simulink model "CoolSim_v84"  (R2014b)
settings: Solver=ode1  StartTime=0.0  StopTime=trun  FixedStep=dtmax  MaxStep=dtmax  MinStep=1e-6  RelTol=1e-4
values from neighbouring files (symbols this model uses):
  aperp_cond = l_cond*gappl_cond - l_cond*densfin_cond*thfin_cond*lfin_cond    (= 0.00397716486616)    [CoolSim_v84_ec_init.m]    (also in CoolSim_v84_mc_init.m)
  apin_txv = 1e-3^2/4*pi    (= 7.85398163397e-07)    [CoolSim_v84_ec_init.m]    (also in CoolSim_v84_mc_init.m)
  area_cabinint = 8.0    (= 8)    [CoolSim_v84_ec_init.m]    (also in CoolSim_v84_mc_init.m)
  area_cabinshell = 4.0    (= 4)    [CoolSim_v84_ec_init.m]    (also in CoolSim_v84_mc_init.m)
  aseat_txv = dball_txv^2/4*pi    (= 7.06858347058e-06)    [CoolSim_v84_ec_init.m]    (also in CoolSim_v84_mc_init.m)
  atop_txv = 400e-6    (= 0.0004)    [CoolSim_v84_ec_init.m]    (also in CoolSim_v84_mc_init.m)
  c08 = -5.8002206e+003    (= -5800.2206)    [CoolSim_v84_ec_init.m]    (also in CoolSim_v84_mc_init.m)
  c09 = 1.3914993    [CoolSim_v84_ec_init.m]    (also in CoolSim_v84_mc_init.m)
  c10 = -4.8640239E-02    (= -0.048640239)    [CoolSim_v84_ec_init.m]    (also in CoolSim_v84_mc_init.m)
  c11 = 4.1764768E-05    (= 4.1764768e-05)    [CoolSim_v84_ec_init.m]    (also in CoolSim_v84_mc_init.m)
  c12 = -1.4452093E-08    (= -1.4452093e-08)    [CoolSim_v84_ec_init.m]    (also in CoolSim_v84_mc_init.m)
  c13 = 6.5459673    [CoolSim_v84_ec_init.m]    (also in CoolSim_v84_mc_init.m)
  c1_comprmech = 0.8728    [CoolSim_v84_ec_init.m]    (also in CoolSim_v84_mc_init.m = 0.9)
  c2_comprmech = 0.1777    [CoolSim_v84_ec_init.m]    (also in CoolSim_v84_mc_init.m = 0)
  cv_air = 719.    (= 719)    [CoolSim_v84_ec_init.m]    (also in CoolSim_v84_mc_init.m)
  deltat = 2e-4    (= 0.0002)    [CoolSim_v84_ec_init.m]    (also in CoolSim_v84_mc_init.m)
  dh_evaptocomp = 0.0    (= 0)    [CoolSim_v84_ec_init.m]    (also in CoolSim_v84_mc_init.m)
  displ_compr = 33e-6    (= 3.3e-05)    [CoolSim_v84_ec_init.m]    (also in CoolSim_v84_mc_init.m = 0.0002)
  dp_blower = [0,  40., 160., 360.]    [CoolSim_v84_ec_init.m]    (also in CoolSim_v84_mc_init.m)
  dp_evaptocomp = 0.0    (= 0)    [CoolSim_v84_ec_init.m]    (also in CoolSim_v84_mc_init.m)
  dpair_cond = 2300.    (= 2300)    [CoolSim_v84_ec_init.m]    (also in CoolSim_v84_mc_init.m)
  dt_evapout = 0.5    [CoolSim_v84_ec_init.m]    (also in CoolSim_v84_mc_init.m)
  dt_thermostat = 0.2    [CoolSim_v84_ec_init.m]    (also in CoolSim_v84_mc_init.m)
  eff_blower = 0.12    [CoolSim_v84_ec_init.m]    (also in CoolSim_v84_mc_init.m)
  eff_fan = 0.15    [CoolSim_v84_ec_init.m]    (also in CoolSim_v84_mc_init.m)
  einitvec_cond1 = 10.*ones(1,nseg_cond1)    [CoolSim_v84_ec_init.m]    (also in CoolSim_v84_mc_init.m)
  einitvec_cond2 = 10.*ones(1,nseg_cond2)    [CoolSim_v84_ec_init.m]    (also in CoolSim_v84_mc_init.m)
  einitvec_evap1 = 10.*ones(1,nseg_evap1)    [CoolSim_v84_ec_init.m]    (also in CoolSim_v84_mc_init.m)
  einitvec_evap2a = 10.*ones(1,nseg_evap2)    [CoolSim_v84_ec_init.m]    (also in CoolSim_v84_mc_init.m)
  einitvec_evap2b = 10.*ones(1,nseg_evap2)    [CoolSim_v84_ec_init.m]    (also in CoolSim_v84_mc_init.m)
  einitvec_evap3 = 10.*ones(1,nseg_evap3)    [CoolSim_v84_ec_init.m]    (also in CoolSim_v84_mc_init.m)
  einitvec_evap4 = 10.*ones(1,nseg_evap4)    [CoolSim_v84_ec_init.m]    (also in CoolSim_v84_mc_init.m)
  f1_blowcontr = -0.7    [CoolSim_v84_ec_init.m]    (also in CoolSim_v84_mc_init.m)
  f1_comprcontr = -0.02    [CoolSim_v84_ec_init.m]    (also in CoolSim_v84_mc_init.m)
  f2_blowcontr = 0.005    [CoolSim_v84_ec_init.m]    (also in CoolSim_v84_mc_init.m)
  f2_comprcontr = 1./6.    (= 0.166666666667)    [CoolSim_v84_ec_init.m]    (also in CoolSim_v84_mc_init.m)
  fp_txv = (psetbulb_txv - pset_txv)*atop_txv - 15e5*aseat_txv    [CoolSim_v84_ec_init.m]    (also in CoolSim_v84_mc_init.m)
  h_lookuphvsps = h1    [CoolSim_v84_ec_init.m]    (also in CoolSim_v84_mc_init.m)
  hmax_heater = 8000.    (= 8000)    [CoolSim_v84_ec_init.m]    (also in CoolSim_v84_mc_init.m)
  htin_enginecomp = 0.0    (= 0)    [CoolSim_v84_ec_init.m]    (also in CoolSim_v84_mc_init.m; point_ec01.m; point_mc01.m)
  htin_solarintvstime = [htin_solarint htin_solarint]    [CoolSim_v84_ec_init.m]    (also in CoolSim_v84_mc_init.m; point_ec01.m = [300. 300.]; point_mc01.m = [300. 300.])
  htin_solarshellvstime = [htin_solarshell htin_solarshell]    [CoolSim_v84_ec_init.m]    (also in CoolSim_v84_mc_init.m; point_ec01.m = [1000. 1000.]; point_mc01.m = [1000. 1000.])
  htrans_cabinint = 25.    (= 25)    [CoolSim_v84_ec_init.m]    (also in CoolSim_v84_mc_init.m)
  htrans_cabinshell = 15.    (= 15)    [CoolSim_v84_ec_init.m]    (also in CoolSim_v84_mc_init.m)
  ifmech = 0.0    (= 0)    [CoolSim_v84_ec_init.m]    (also in CoolSim_v84_mc_init.m = 1)
  iinitvec_cond1 = 0.0*ones(1,nseg_cond1+1)    [CoolSim_v84_ec_init.m]    (also in CoolSim_v84_mc_init.m)
  iinitvec_cond2 = 0.0*ones(1,nseg_cond2+1)    [CoolSim_v84_ec_init.m]    (also in CoolSim_v84_mc_init.m)
  iinitvec_evap1 = 0.0*ones(1,nseg_evap1+1)    [CoolSim_v84_ec_init.m]    (also in CoolSim_v84_mc_init.m)
  iinitvec_evap2a = 0.0*ones(1,nseg_evap2+1)    [CoolSim_v84_ec_init.m]    (also in CoolSim_v84_mc_init.m)
  iinitvec_evap2b = 0.0*ones(1,nseg_evap2+1)    [CoolSim_v84_ec_init.m]    (also in CoolSim_v84_mc_init.m)
  iinitvec_evap3 = 0.0*ones(1,nseg_evap3+1)    [CoolSim_v84_ec_init.m]    (also in CoolSim_v84_mc_init.m)
  iinitvec_evap4 = 0.0*ones(1,nseg_evap4+1)    [CoolSim_v84_ec_init.m]    (also in CoolSim_v84_mc_init.m)
  init_memrestart = 2250.    (= 2250)    [CoolSim_v84_ec_init.m]    (also in CoolSim_v84_mc_init.m; reinit.m = memrestart(n,2))
  init_picontr1 = 0.23    [CoolSim_v84_ec_init.m]    (also in CoolSim_v84_mc_init.m; reinit.m = picontr1(n,2))
  init_picontr2 = 0.32    [CoolSim_v84_ec_init.m]    (also in CoolSim_v84_mc_init.m; reinit.m = picontr2(n,2))
  iseff_rpm_pr = [0.650   0.728   0.717   0.655   0.569;     0.570   0.682   0.700   0.637   0.536;     0.460   0.590   0.650   0.600   0.493;     0.290   0.496   0.618   0.575   0.450]    [CoolSim_v84_ec_init.m]    (also in CoolSim_v84_mc_init.m = [0.8490    0.8490    0.7829    0.7409    0.7065    0.6802   )
  k_cabinleakin = 1e-4    (= 0.0001)    [CoolSim_v84_ec_init.m]    (also in CoolSim_v84_mc_init.m)
  k_cabinleakout = 4e-4    (= 0.0004)    [CoolSim_v84_ec_init.m]    (also in CoolSim_v84_mc_init.m)
  k_ram = 0.1    [CoolSim_v84_ec_init.m]    (also in CoolSim_v84_mc_init.m)
  l_cabinsurf = 2.0    (= 2)    [CoolSim_v84_ec_init.m]    (also in CoolSim_v84_mc_init.m)
  md_comprmax = rpm_max/60.*displ_compr*0.975*27.8    (= 0.10435425)    [CoolSim_v84_ec_init.m]    (also in CoolSim_v84_mc_init.m = 0.63245)
  minitvec_cond1 = 1e-4*ones(1,nseg_cond1)    [CoolSim_v84_ec_init.m]    (also in CoolSim_v84_mc_init.m)
  minitvec_cond2 = 1e-4*ones(1,nseg_cond2)    [CoolSim_v84_ec_init.m]    (also in CoolSim_v84_mc_init.m)
  minitvec_evap1 = 1e-4*ones(1,nseg_evap1)    [CoolSim_v84_ec_init.m]    (also in CoolSim_v84_mc_init.m)
  minitvec_evap2a = 1e-4*ones(1,nseg_evap2)    [CoolSim_v84_ec_init.m]    (also in CoolSim_v84_mc_init.m)
  minitvec_evap2b = 1e-4*ones(1,nseg_evap2)    [CoolSim_v84_ec_init.m]    (also in CoolSim_v84_mc_init.m)
  minitvec_evap3 = 1e-4*ones(1,nseg_evap3)    [CoolSim_v84_ec_init.m]    (also in CoolSim_v84_mc_init.m)
  minitvec_evap4 = 1e-4*ones(1,nseg_evap4)    [CoolSim_v84_ec_init.m]    (also in CoolSim_v84_mc_init.m)
  mrefr_outrate = 0.2    [CoolSim_v84_ec_init.m]    (also in CoolSim_v84_mc_init.m)
  mrefr_targ = 0.48    [CoolSim_v84_ec_init.m]    (also in CoolSim_v84_mc_init.m)
  nc1 = 35.    (= 35)    [CoolSim_v84_ec_init.m]    (also in CoolSim_v84_mc_init.m)
  nc2 = 9.0    (= 9)    [CoolSim_v84_ec_init.m]    (also in CoolSim_v84_mc_init.m)
  ne1 = 7.    (= 7)    [CoolSim_v84_ec_init.m]    (also in CoolSim_v84_mc_init.m)
  ne2a = 5.    (= 5)    [CoolSim_v84_ec_init.m]    (also in CoolSim_v84_mc_init.m)
  ne2b = 15.    (= 15)    [CoolSim_v84_ec_init.m]    (also in CoolSim_v84_mc_init.m)
  ne3 = 12.    (= 12)    [CoolSim_v84_ec_init.m]    (also in CoolSim_v84_mc_init.m)
  ne4 = 15.    (= 15)    [CoolSim_v84_ec_init.m]    (also in CoolSim_v84_mc_init.m)
  onoff_fanonoffvstime = [1  1]    [CoolSim_v84_ec_init.m]    (also in CoolSim_v84_mc_init.m; point_ec01.m; point_mc01.m)
  onoffinit_cabin = 1.0    (= 1)    [CoolSim_v84_ec_init.m]    (also in CoolSim_v84_mc_init.m; reinit.m = onoff_cabin(n,2))
  onoffinit_evap = 1.0    (= 1)    [CoolSim_v84_ec_init.m]    (also in CoolSim_v84_mc_init.m; reinit.m = onoff_evap(n,2))
  p_ambient = 1.013e5    (= 101300)    [CoolSim_v84_ec_init.m]    (also in CoolSim_v84_mc_init.m)
  p_ambvstime = [p_ambient p_ambient]    [CoolSim_v84_ec_init.m]    (also in CoolSim_v84_mc_init.m; point_ec01.m = [101300. 101300.]; point_mc01.m = [101300. 101300.])
  p_lookup_tsatvsp = psat*1e5    [CoolSim_v84_ec_init.m]    (also in CoolSim_v84_mc_init.m)
  r_h2o = 461.5043    [CoolSim_v84_ec_init.m]    (also in CoolSim_v84_mc_init.m)
  rair = 287.    (= 287)    [CoolSim_v84_ec_init.m]    (also in CoolSim_v84_mc_init.m)
  rate_txv = 35e3    (= 35000)    [CoolSim_v84_ec_init.m]    (also in CoolSim_v84_mc_init.m)
  ratio_compr = 1.37    [CoolSim_v84_ec_init.m]    (also in CoolSim_v84_mc_init.m)
  rh_ambvstime = [rh_ambient rh_ambient]    [CoolSim_v84_ec_init.m]    (also in CoolSim_v84_mc_init.m; point_ec01.m = [50. 50.]; point_mc01.m = [50. 50.])
  rpm_max = 7000.    (= 7000)    [CoolSim_v84_ec_init.m]    (also in CoolSim_v84_mc_init.m)
  rpm_minmaxrat = 1500./7000.    (= 0.214285714286)    [CoolSim_v84_ec_init.m]    (also in CoolSim_v84_mc_init.m)
  rpm_rpmvstime = [1600,  1600]    [CoolSim_v84_ec_init.m]    (also in CoolSim_v84_mc_init.m; point_mc01.m)
  rpm_switchoff = rpm_max*rpm_minmaxrat*1.01    (= 1515)    [CoolSim_v84_ec_init.m]    (also in CoolSim_v84_mc_init.m)
  s_txv = 0.8e-3    (= 0.0008)    [CoolSim_v84_ec_init.m]    (also in CoolSim_v84_mc_init.m)
  scfm_blower = [0, 100., 200., 300.]    [CoolSim_v84_ec_init.m]    (also in CoolSim_v84_mc_init.m)
  set_steadystate = 0.0    (= 0)    [CoolSim_v84_ec_init.m]    (also in CoolSim_v84_mc_init.m)
  setting_blend = 0.0    (= 0)    [CoolSim_v84_ec_init.m]    (also in CoolSim_v84_mc_init.m; point_mc01.m)
  setting_blower = 3.0    (= 3)    [CoolSim_v84_ec_init.m]    (also in CoolSim_v84_mc_init.m; point_mc01.m)
  setting_recirc = -1.0    (= -1)    [CoolSim_v84_ec_init.m]    (also in CoolSim_v84_mc_init.m; point_mc01.m = 0.95)
  shape_cabinsurf = 0.5    [CoolSim_v84_ec_init.m]    (also in CoolSim_v84_mc_init.m)
  smin_txv = 1e-6    (= 1e-06)    [CoolSim_v84_ec_init.m]    (also in CoolSim_v84_mc_init.m)
  t_ambvstime = [t_ambient t_ambient]    [CoolSim_v84_ec_init.m]    (also in CoolSim_v84_mc_init.m; point_ec01.m = [303.16 303.16]; point_mc01.m = [303.16 303.16])
  t_lookup_tsatvsp = t1    [CoolSim_v84_ec_init.m]    (also in CoolSim_v84_mc_init.m)
  tairevapout_limit = 274.    (= 274)    [CoolSim_v84_ec_init.m]    (also in CoolSim_v84_mc_init.m)
  tairin_cond = 303.16    [CoolSim_v84_ec_init.m]    (also in CoolSim_v84_mc_init.m; point_ec01.m; point_mc01.m)
  tbulbinit_txv = 273.0    (= 273)    [CoolSim_v84_ec_init.m]    (also in CoolSim_v84_mc_init.m; reinit.m = tbulb_txv(n,2))
  tchar_txv = 0.1    [CoolSim_v84_ec_init.m]    (also in CoolSim_v84_mc_init.m)
  tdel_cycling = 5.0    (= 5)    [CoolSim_v84_ec_init.m]    (also in CoolSim_v84_mc_init.m)
  tdelinit_cycling = 1.0    (= 1)    [CoolSim_v84_ec_init.m]    (also in CoolSim_v84_mc_init.m; reinit.m = tdel_cycling1(n,2))
  tevap_target = 273.16+3.0    (= 276.16)    [CoolSim_v84_ec_init.m]    (also in CoolSim_v84_mc_init.m)
  thmass_cabinint = 2e5    (= 200000)    [CoolSim_v84_ec_init.m]    (also in CoolSim_v84_mc_init.m)
  thmass_cabinshell = 1e5    (= 100000)    [CoolSim_v84_ec_init.m]    (also in CoolSim_v84_mc_init.m)
  time0 = 0.0    (= 0)    [CoolSim_v84_ec_init.m]    (also in CoolSim_v84_mc_init.m; reinit.m = time11(n,2))
  time_ambvstime = [0 1e5]    [CoolSim_v84_ec_init.m]    (also in CoolSim_v84_mc_init.m; point_ec01.m; point_mc01.m)
  time_fanonoffvstime = [0 1e5]    [CoolSim_v84_ec_init.m]    (also in CoolSim_v84_mc_init.m; point_ec01.m; point_mc01.m)
  time_rpmvstime = [0,    10000]    [CoolSim_v84_ec_init.m]    (also in CoolSim_v84_mc_init.m; point_mc01.m)
  time_solarintvstime = [0 1e5]    [CoolSim_v84_ec_init.m]    (also in CoolSim_v84_mc_init.m; point_ec01.m; point_mc01.m)
  time_solarshellvstime = [0 1e5]    [CoolSim_v84_ec_init.m]    (also in CoolSim_v84_mc_init.m; point_ec01.m; point_mc01.m)
  time_velvstime = [0 1e5]    [CoolSim_v84_ec_init.m]    (also in CoolSim_v84_mc_init.m; point_ec01.m; point_mc01.m)
  tinit_cabinint = 313.16    [CoolSim_v84_ec_init.m]    (also in CoolSim_v84_mc_init.m; point_ec01.m; point_mc01.m; reinit.m = t_cabinint(n,2))
  tinit_cabinshell = 308.16    [CoolSim_v84_ec_init.m]    (also in CoolSim_v84_mc_init.m; point_ec01.m; point_mc01.m; reinit.m = t_cabinshell(n,2))
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undefined symbols (not defined in the file or in its folder): nseg
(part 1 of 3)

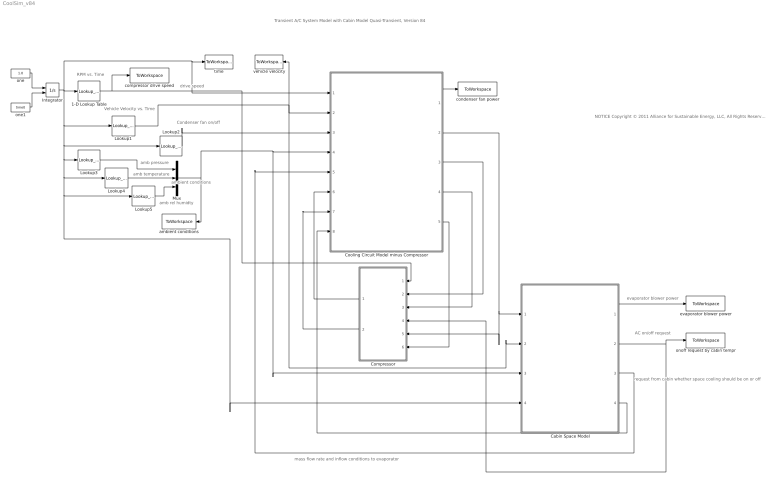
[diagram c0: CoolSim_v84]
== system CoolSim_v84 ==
  note: drive speed
  note: evaporator blower power
  note: RPM vs. Time
  note: Transient A/C System Model with Cabin Model Quasi-Transient, Version 84
  note: ambient conditions
  note: Vehicle Velocity vs. Time
  note: Condenser fan on/off
  note: amb pressure
  note: amb temperature
  note: amb rel humidty
  note: request from cabin whether space cooling should be on or off
  note: mass flow rate and inflow conditions to evaporator
  note: AC on/off request
  note: NOTICE Copyright © 2011 Alliance for Sustainable Energy, LLC, All Rights Reserved The CoolSim software (“ Software”) is being provided for internal, noncommercial purposes only and shall not be re-distributed. This Software was produced by Alliance for Sustainable Energy, LLC, (“Contactor”) under Contract No. DE-AC36-08GO28308 with the Department of Energy (“DOE”). For five (5) years from the date permission to assert copyright is obtained, the Government is granted for itself and others acting on its behalf a nonexclusive, paid-up, irrevocable worldwide license in this Software to reproduce, prepare derivative works, and perform publicly and display publicly, by or on behalf of the Government. There is provision for the possible extension of the term of this license. Subsequent to that period or any extension granted, the Government is granted for itself and others acting on its behalf a nonexclusive, paid-up, irrevocable worldwide license in this Software to reproduce, prepare derivative works, distribute copies to the public, perform publicly and display publicly, and to permit others to do so. The specific term of the license can be identified by inquiry made to Contractor or DOE. NEITHER THE UNITED STATES NOR THE UNITED STATES DEPARTMENT OF ENERGY, NOR ANY OF THEIR EMPLOYEES, MAKES ANY WARRANTY, EXPRESS OR IMPLIED, OR ASSUMES ANY LEGAL LIABILITY OR RESPONSIBILITY FOR THE ACCURACY, COMPLETENESS, OR USEFULNESS OF ANY DATA, APPARATUS, PRODUCT, OR PROCESS DISCLOSED, OR REPRESENTS THAT ITS USE WOULD NOT INFRINGE PRIVATELY OWNED RIGHTS.THIS SOFTWARE IS PROVIDED BY THE CONTRACTOR "AS IS" AND ANY EXPRESS OR IMPLIED WARRANTIES, INCLUDING BUT NOT LIMITED TO, THE IMPLIED WARRANTIES OF MERCHANTABILITY AND FITNESS FOR A PARTICULAR PURPOSE ARE EXPRESSLY DISCLAIMED. IN NO EVENT SHALL THE CONTRACTOR OR THE U.S. GOVERNMENT BE LIABLE FOR ANY SPECIAL, INDIRECT OR CONSEQUENTIAL DAMAGES OR ANY DAMAGES WHATSOEVER, INCLUDING BUT NOT LIMITED TO CLAIMS ASSOCIATED WITH THE LOSS OF DATA 
  1-D Lookup Table : Lookup_n-D  NumberOfTableDimensions=1  BreakpointsForDimension1=time_rpmvstime  Table=rpm_rpmvstime  RndMeth=Simplest
  Cabin Space Model : Subsystem
  Compressor : Subsystem
  Cooling Circuit Model minus Compressor : Subsystem
  Integrator : Integrator  InitialConditionSource=external
  Lookup1 : Lookup_n-D  NumberOfTableDimensions=1  BreakpointsForDimension1=time_velvstime  Table=vel_velvstime  RndMeth=Simplest
  Lookup2 : Lookup_n-D  NumberOfTableDimensions=1  BreakpointsForDimension1=time_fanonoffvstime  Table=onoff_fanonoffvstime  RndMeth=Simplest
  Lookup3 : Lookup_n-D  NumberOfTableDimensions=1  BreakpointsForDimension1=time_ambvstime  Table=p_ambvstime  RndMeth=Simplest
  Lookup4 : Lookup_n-D  NumberOfTableDimensions=1  BreakpointsForDimension1=time_ambvstime  Table=t_ambvstime  RndMeth=Simplest
  Lookup5 : Lookup_n-D  NumberOfTableDimensions=1  BreakpointsForDimension1=time_ambvstime  Table=rh_ambvstime  RndMeth=Simplest
  Mux : Mux  Inputs=3
  ambient conditions : ToWorkspace  VariableName=ambient  SampleTime=-1
  compressor drive speed : ToWorkspace  VariableName=rpm_drive1  SampleTime=-1
  condenser fan power : ToWorkspace  VariableName=power_condfan  SampleTime=-1
  evaporator blower power : ToWorkspace  VariableName=power_blower  SampleTime=-1
  one : Constant  Value=1.0
  one1 : Constant  Value=time0
  onoff request by cabin tempr : ToWorkspace  VariableName=onoff_cabin1  SampleTime=-1
  time : ToWorkspace  VariableName=time1  SampleTime=-1
  vehicle velocity : ToWorkspace  VariableName=velvehicle  SampleTime=-1
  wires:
  1-D Lookup Table/1 -> compressor drive speed/1, Compressor/1(rpm)
  Integrator/1 -> 1-D Lookup Table/1, Lookup1/1, Lookup4/1, Lookup5/1, Cabin Space Model/4(time1), Lookup3/1, Lookup2/1, time/1, Cooling Circuit Model minus Compressor/1(time1)
  one/1 -> Integrator/1
  one1/1 -> Integrator/2
  Lookup1/1 -> vehicle velocity/1, Cabin Space Model/2(vel_vechicle), Cooling Circuit Model minus Compressor/2(vel_vehicle)
  Mux/1 -> ambient conditions/1, Cooling Circuit Model minus Compressor/4(ambient), Cabin Space Model/3(ambient)
  Lookup3/1 -> Mux/1
  Lookup4/1 -> Mux/2
  Lookup5/1 -> Mux/3
  Lookup2/1 -> Cooling Circuit Model minus Compressor/3(fan)
  Cabin Space Model/1(pw_blower) -> evaporator blower power/1
  Cooling Circuit Model minus Compressor/1(power_cond_fan) -> condenser fan power/1
  Cooling Circuit Model minus Compressor/2(flowout_evap) -> Cabin Space Model/1(flowout_evap), Compressor/5(tevapout)
  Cabin Space Model/2(AC_request) -> onoff request by cabin tempr/1, Compressor/4(AC_request)
  Cabin Space Model/3(airevapin) -> Cooling Circuit Model minus Compressor/5(airinevap)
  Compressor/2(qd) -> Cooling Circuit Model minus Compressor/7(qdcompr)
  Cooling Circuit Model minus Compressor/3(pucompr) -> Compressor/2(ptrhu)
  Cooling Circuit Model minus Compressor/4(pdcompr) -> Compressor/3(ptrhd)
  Compressor/1(qu) -> Cooling Circuit Model minus Compressor/6(qucompr)
  Cabin Space Model/4(ambextras) -> Cooling Circuit Model minus Compressor/8(ambextras)
  Cooling Circuit Model minus Compressor/5(twallevap) -> Compressor/6(twallevap)

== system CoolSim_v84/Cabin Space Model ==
  note: mass flow rate from cabin to blower
  note: all air flow to blower
  note: total air inflow to cabin
  note: blower power use
  note: md, tempr, RH out evap
  note: fraction reheat request
  note: rho, h, ah ambient
  note: md, hd, ah
  note: md, hd, ah
  note: air mass flow rate to blower from cabin
  note: changed for mc02!!!
  flowout_evap : Inport
  vel_vechicle : Inport  Port=2
  ambient : Inport  Port=3
  time1 : Inport  Port=4
  airmix_volume02 CABIN : Subsystem
  cabin properties : ToWorkspace  VariableName=pcabin  SampleTime=-1
  calculate cabin heat load : Subsystem
  calculate air inflow to evap : Subsystem
  calculate cabin air inflow : Subsystem
  calculate desired settings : Subsystem
  calculate outflow from cabin : Subsystem
  evap airflow recirculated portion : ToWorkspace  VariableName=recirc  SampleTime=-1
  save data for reninitialization : Subsystem
  select pres : Fcn  Expr=u(1)
  zeros1 : Constant  Value=[vol_cabin, 0.0]
  pw_blower : Outport
  AC_request : Outport  Port=2
  airevapin : Outport  Port=3
  ambextras : Outport  Port=4
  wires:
  flowout_evap/1 -> calculate cabin air inflow/1(evapout)
  vel_vechicle/1 -> calculate cabin heat load/1(vveh)
  calculate desired settings/3(Blower) -> calculate air inflow to evap/2(blower)
  zeros1/1 -> airmix_volume02 CABIN/2("V, dVdt")
  airmix_volume02 CABIN/1(ptrh_mix) -> calculate desired settings/1(cabin), calculate air inflow to evap/1(cabin), calculate outflow from cabin/1(cabin), calculate cabin heat load/3(cabin), select pres/1, [pcabin], cabin properties/1
  calculate cabin air inflow/1(inflow) -> airmix_volume02 CABIN/1(qu)
  calculate outflow from cabin/1(outflow) -> airmix_volume02 CABIN/4(qd)
  ambient/1 -> calculate cabin heat load/2(ambient), calculate cabin air inflow/2(ambient), calculate outflow from cabin/2(ambient), calculate desired settings/2(ambient)
  calculate cabin heat load/1(htout) -> airmix_volume02 CABIN/3(Hout)
  calculate air inflow to evap/2(airinevap) -> airevapin/1
  calculate air inflow to evap/3(toevap) -> calculate outflow from cabin/3(toevap)
  calculate desired settings/4(Recirc) -> calculate air inflow to evap/3(recirc), evap airflow recirculated portion/1
  calculate desired settings/2(AC_on) -> AC_request/1
  calculate air inflow to evap/1(pwblower) -> pw_blower/1
  select pres/1 -> calculate cabin air inflow/3(pcabin)
  calculate desired settings/1(blend) -> calculate cabin air inflow/4(blend)
  [ambextras] -> calculate air inflow to evap/4(ambient), ambextras/1
  time1/1 -> calculate cabin heat load/4(time1)

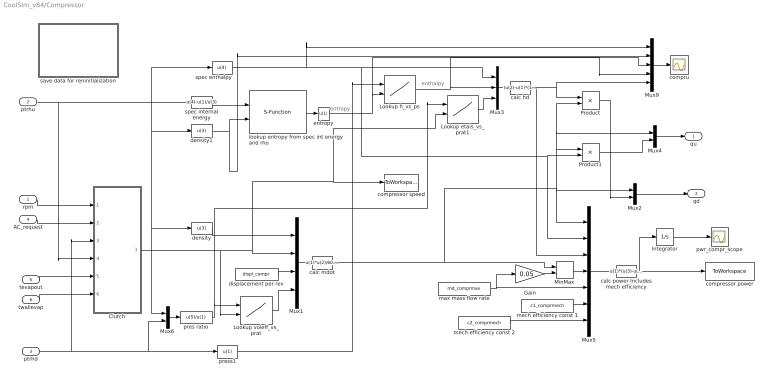
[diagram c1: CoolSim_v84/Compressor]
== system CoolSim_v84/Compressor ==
  note: enthalpy
  note: entropy
  rpm : Inport
  ptrhu : Inport  Port=2
  ptrhd : Inport  Port=3
  AC_request : Inport  Port=4
  tevapout : Inport  Port=5
  twallevap : Inport  Port=6
  Clutch : Subsystem
  Gain : Gain  Gain=0.05
  Integrator : Integrator
  Lookup etais_vs_prat1 : Lookup2D  RowIndex=voleff_prs  ColumnIndex=voleff_rpms  Table=iseff_rpm_pr  LookUpMeth=Interpolation-Use End Values
  Lookup h_vs_ps : Lookup2D  RowIndex=p_lookuphvsps  ColumnIndex=s_lookuphvsps  Table=h_lookuphvsps
  Lookup voleff_vs_prat : Lookup2D  RowIndex=voleff_prs  ColumnIndex=voleff_rpms  Table=voleff_rpm_pr  LookUpMeth=Interpolation-Use End Values
  MinMax : MinMax  Function=max  Inputs=2
  Mux1 : Mux
  Mux2 : Mux  Inputs=2
  Mux3 : Mux  Inputs=3
  Mux4 : Mux  Inputs=2
  Mux5 : Mux  Inputs=7
  Mux6 : Mux  Inputs=2
  Mux9 : Mux  Inputs=5
  Product : Product
  Product1 : Product
  calc hd : Fcn  Expr=(u(2)-u(1)*(1.0-u(3)))/u(3)
  calc mdot : Fcn  Expr=u(1)*u(2)/60.*u(3)*u(4)
  calc power Includes mech efficiency : Fcn  Expr=u(1)*(u(3)-u(2)) / (u(6)+u(7)*log( u(4)/u(5)))
  compressor power : ToWorkspace  VariableName=power_compr  SampleTime=-1
  compressor speed : ToWorkspace  VariableName=rpm_compr  SampleTime=-1
  compru : Scope
  density : Fcn  Expr=u(3)
  density1 : Fcn  Expr=u(3)
  displacement per rev : Constant  Value=displ_compr
  entropy : Fcn  Expr=u(1)
  lookup entropy from spec int energy and rho : S-Function  FunctionName=lookup_s_vs_urho  Parameters=1  EnableBusSupport=off
  max mass flow rate : Constant  Value=md_comprmax
  mech efficiency const 1 : Constant  Value=c1_comprmech
  mech efficiency const 2 : Constant  Value=c2_comprmech
  pres ratio : Fcn  Expr=u(5)/u(1)
  press1 : Fcn  Expr=u(1)
  pwr_compr_scope : Scope
  save data for reninitialization : Subsystem
  spec enthalpy : Fcn  Expr=u(4)
  spec internal energy : Fcn  Expr=u(4)-u(1)/u(3)
  qu : Outport
  qd : Outport  Port=2
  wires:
  ptrhu/1 -> Clutch/4(pucompr), spec internal energy/1, spec enthalpy/1, density/1, Mux6/1, density1/1
  density/1 -> Mux1/1
  Clutch/1(rpm) -> Mux1/2, compressor speed/1, Lookup etais_vs_prat1/2, Lookup voleff_vs_prat/2
  displacement per rev/1 -> Mux1/3
  Mux1/1 -> calc mdot/1
  ptrhd/1 -> press1/1, Mux6/2, Clutch/3(pdcompr)
  press1/1 -> Lookup h_vs_ps/1
  spec enthalpy/1 -> Mux3/1, Product1/2, Mux5/2, Mux9/1
  Lookup h_vs_ps/1 -> Mux9/4, Mux3/2
  Lookup etais_vs_prat1/1 -> Mux3/3
  Mux3/1 -> calc hd/1
  calc hd/1 -> Mux5/3, Product/1, Mux9/5
  calc mdot/1 -> Mux2/1, Product/2, Mux4/1, Product1/1, Mux5/1, MinMax/1
  Product/1 -> Mux2/2
  Mux2/1 -> qd/1
  Mux4/1 -> qu/1
  Product1/1 -> Mux4/2
  entropy/1 -> Lookup h_vs_ps/2, Mux9/3
  Mux6/1 -> pres ratio/1
  pres ratio/1 -> Lookup voleff_vs_prat/1, Lookup etais_vs_prat1/1
  Lookup voleff_vs_prat/1 -> Mux1/4
  lookup entropy from spec int energy and rho/1 -> entropy/1
  spec internal energy/1 -> lookup entropy from spec int energy and rho/1
  density1/1 -> lookup entropy from spec int energy and rho/2, Mux9/2
  Mux9/1 -> compru/1
  calc power Includes mech efficiency/1 -> Integrator/1, compressor power/1
  Integrator/1 -> pwr_compr_scope/1
  Mux5/1 -> calc power Includes mech efficiency/1
  mech efficiency const 2/1 -> Mux5/7
  max mass flow rate/1 -> Gain/1, Mux5/5
  Gain/1 -> MinMax/2
  MinMax/1 -> Mux5/4
  mech efficiency const 1/1 -> Mux5/6
  AC_request/1 -> Clutch/2(aconoff)
  rpm/1 -> Clutch/1(driverpm)
  tevapout/1 -> Clutch/5(tevapout)
  twallevap/1 -> Clutch/6(twallevap)

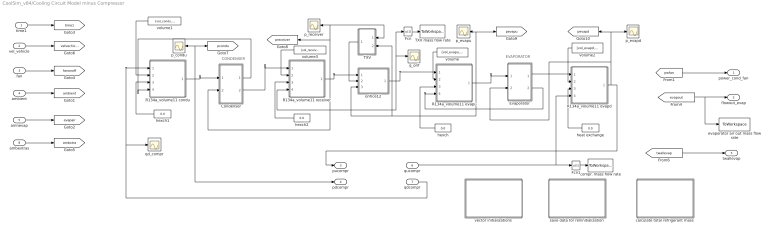
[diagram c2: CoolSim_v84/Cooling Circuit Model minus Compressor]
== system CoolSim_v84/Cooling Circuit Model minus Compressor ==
  note: CONDENSER
  note: EVAPORATOR
  time1 : Inport
  vel_vehicle : Inport  Port=2
  fan : Inport  Port=3
  ambient : Inport  Port=4
  airinevap : Inport  Port=5
  qucompr : Inport  Port=6
  qdcompr : Inport  Port=7
  ambextras : Inport  Port=8
  Condenser : Subsystem
  Evaporator : Subsystem
  Fcn : Fcn  Expr=u(1)
  Fcn1 : Fcn  Expr=u(1)
  R134a_volume11 condu : Subsystem
  R134a_volume11 evapd : Subsystem
  R134a_volume11 evapu : Subsystem
  R134a_volume11 receiver : Subsystem
  TXV : Subsystem
  TXV mass flow rate : ToWorkspace  VariableName=qorif  SampleTime=-1
  calculate total refrigerant mass : Subsystem
  compr. mass flow rate : ToWorkspace  VariableName=qcompr  SampleTime=-1
  evaporator air out mass flow rate : ToWorkspace  VariableName=mdaout_evap  SampleTime=-1
  heat exchange : Constant  Value=0.0
  hexch : Constant  Value=0.0
  hexch1 : Constant  Value=0.0
  hexch2 : Constant  Value=0.0
  orifice12 : Subsystem
  p_condu : Scope
  p_evapd : Scope
  p_evapu : Scope
  p_receiver : Scope
  q_orif : Scope
  qd_compr : Scope
  save data for reninitialization : Subsystem
  vector initializations : Subsystem
  volume : Constant  Value=[vol_evapu, 0]
  volume1 : Constant  Value=[vol_condu, 0]
  volume2 : Constant  Value=[vol_evapd, 0]
  volume3 : Constant  Value=[vol_receiver, 0]
  power_cond_fan : Outport
  flowout_evap : Outport  Port=2
  pucompr : Outport  Port=3
  pdcompr : Outport  Port=4
  twallevap : Outport  Port=5
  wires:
  R134a_volume11 condu/1(ptrh_mix) -> Condenser/1(ptrhu), p_condu/1, [pcondu], pdcompr/1
  orifice12/1(qmh) -> R134a_volume11 evapu/1(qu), q_orif/1, Fcn/1, R134a_volume11 receiver/4(qd)
  volume/1 -> R134a_volume11 evapu/2("V, dVdt")
  qucompr/1 -> R134a_volume11 evapd/4(qd), Fcn1/1
  volume1/1 -> R134a_volume11 condu/2("V, dVdt")
  qdcompr/1 -> R134a_volume11 condu/1(qu), qd_compr/1
  TXV/1(afr) -> orifice12/2(afrac)
  volume2/1 -> R134a_volume11 evapd/2("V, dVdt")
  R134a_volume11 evapd/1(ptrh_mix) -> Evaporator/2(ptrhd), p_evapd/1, [pevapd], pucompr/1
  heat exchange/1 -> R134a_volume11 evapd/3(Hout)
  R134a_volume11 evapu/1(ptrh_mix) -> Evaporator/1(ptrhu), p_evapu/1, [pevapu], orifice12/3(pTrhd), TXV/2(pd)
  hexch/1 -> R134a_volume11 evapu/3(Hout)
  R134a_volume11 receiver/1(ptrh_mix) -> orifice12/1(pTrhu), p_receiver/1, TXV/1(pu), [preceiver], Condenser/2(ptrhd)
  Condenser/1(qmhu) -> R134a_volume11 condu/4(qd)
  Condenser/2(qmhd) -> R134a_volume11 receiver/1(qu)
  volume3/1 -> R134a_volume11 receiver/2("V, dVdt")
  hexch2/1 -> R134a_volume11 receiver/3(Hout)
  hexch1/1 -> R134a_volume11 condu/3(Hout)
  Evaporator/1(qmhd) -> R134a_volume11 evapd/1(qu)
  Evaporator/2(qmhu) -> R134a_volume11 evapu/4(qd)
  [pwfan] -> power_cond_fan/1
  [evapout] -> flowout_evap/1, evaporator air out mass flow rate/1
  vel_vehicle/1 -> [velvechicle]
  ambient/1 -> [ambient]
  airinevap/1 -> [evapair]
  Fcn/1 -> TXV mass flow rate/1
  Fcn1/1 -> compr. mass flow rate/1
  fan/1 -> [fanonoff]
  ambextras/1 -> [ambxtra]
  [twallevap] -> twallevap/1
  time1/1 -> [time1]

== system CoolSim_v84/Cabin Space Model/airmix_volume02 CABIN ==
  note: p, T, rho, h, mh2o, rh, ah
  note: md_in, hd_in, ah_in
  note: md_out, hd_out, ah_out
  note: heat energy outflow rate
  note: volume, and time derivative of volume
  qu : Inport
  "V, dVdt" : Inport  Port=2
  Hout : Inport  Port=3
  qd : Inport  Port=4
  S-Function : S-Function  FunctionName=airmix_volume04  Parameters=vol0, mh2o0, p0, t0, rh0  EnableBusSupport=off
  ptrh_mix : Outport
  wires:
  qd/1 -> S-Function/4
  Hout/1 -> S-Function/3
  "V, dVdt"/1 -> S-Function/2
  S-Function/1 -> ptrh_mix/1
  qu/1 -> S-Function/1

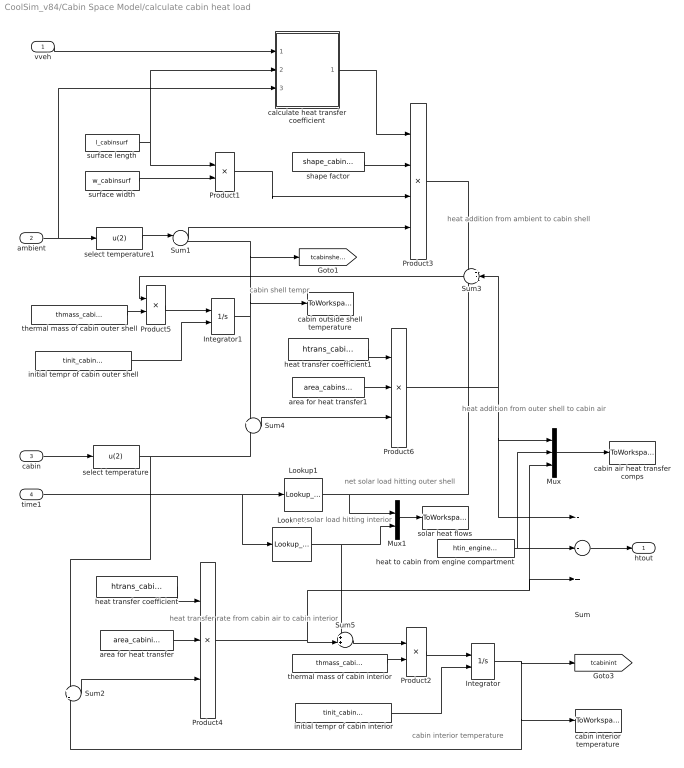
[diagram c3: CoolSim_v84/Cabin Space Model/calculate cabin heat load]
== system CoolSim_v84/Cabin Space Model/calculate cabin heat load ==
  note: heat addition from outer shell to cabin air
  note: cabin interior temperature
  note: heat transfer rate from cabin air to cabin interior
  note: cabin shell tempr
  note: heat addition from ambient to cabin shell
  note: net solar load hitting interior
  note: net solar load hitting outer shell
  vveh : Inport
  ambient : Inport  Port=2
  cabin : Inport  Port=3
  time1 : Inport  Port=4
  Integrator : Integrator  InitialConditionSource=external
  Integrator1 : Integrator  InitialConditionSource=external
  Lookup1 : Lookup_n-D  NumberOfTableDimensions=1  BreakpointsForDimension1=time_solarshellvstime  Table=htin_solarshellvstime  RndMeth=Simplest
  Lookup2 : Lookup_n-D  NumberOfTableDimensions=1  BreakpointsForDimension1=time_solarintvstime  Table=htin_solarintvstime  RndMeth=Simplest
  Mux : Mux  Inputs=3
  Mux1 : Mux  Inputs=2
  Product1 : Product
  Product2 : Product  Inputs=*/
  Product3 : Product  Inputs=4
  Product4 : Product  Inputs=3
  Product5 : Product  Inputs=*/
  Product6 : Product  Inputs=3
  Sum : Sum  Inputs=--+
  Sum1 : Sum  Inputs=|+-
  Sum2 : Sum  Inputs=+|-
  Sum3 : Sum  Inputs=+-+
  Sum4 : Sum  Inputs=+|-
  Sum5 : Sum  Inputs=++|
  area for heat transfer : Constant  Value=area_cabinint
  area for heat transfer1 : Constant  Value=area_cabinshell
  cabin air heat transfer comps : ToWorkspace  VariableName=hx_cabinair  SampleTime=-1
  cabin interior temperature : ToWorkspace  VariableName=tcabinint  SampleTime=-1
  cabin outside shell temperature : ToWorkspace  VariableName=tcabinshell  SampleTime=-1
  calculate heat transfer coefficient : Subsystem
  heat to cabin from engine compartment : Constant  Value=htin_enginecomp
  heat transfer coefficient : Constant  Value=htrans_cabinint
  heat transfer coefficient1 : Constant  Value=htrans_cabinshell
  initial tempr of cabin interior : Constant  Value=tinit_cabinint
  initial tempr of cabin outer shell : Constant  Value=tinit_cabinshell
  select temperature : Fcn  Expr=u(2)
  select temperature1 : Fcn  Expr=u(2)
  shape factor : Constant  Value=shape_cabinsurf
  solar heat flows : ToWorkspace  VariableName=htinsolar  SampleTime=-1
  surface length : Constant  Value=l_cabinsurf
  surface width : Constant  Value=w_cabinsurf
  thermal mass of cabin interior : Constant  Value=thmass_cabinint
  thermal mass of cabin outer shell : Constant  Value=thmass_cabinshell
  htout : Outport
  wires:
  ambient/1 -> select temperature1/1, calculate heat transfer coefficient/3(amb)
  cabin/1 -> select temperature/1
  select temperature1/1 -> Sum1/1
  select temperature/1 -> Sum2/1, Sum4/2
  heat to cabin from engine compartment/1 -> Sum/2, Mux/2
  Product3/1 -> Sum3/1
  Sum/1 -> htout/1
  shape factor/1 -> Product3/2
  vveh/1 -> calculate heat transfer coefficient/1(vveh)
  calculate heat transfer coefficient/1(h) -> Product3/1
  Product1/1 -> Product3/3
  surface width/1 -> Product1/2
  surface length/1 -> Product1/1, calculate heat transfer coefficient/2(Ingth)
  Integrator/1 -> [tcabinint], Sum2/2, cabin interior temperature/1
  Product2/1 -> Integrator/1
  thermal mass of cabin interior/1 -> Product2/2
  initial tempr of cabin interior/1 -> Integrator/2
  Sum2/1 -> Product4/3
  area for heat transfer/1 -> Product4/2
  heat transfer coefficient/1 -> Product4/1
  Sum1/1 -> Product3/4
  Product5/1 -> Integrator1/1
  thermal mass of cabin outer shell/1 -> Product5/2
  initial tempr of cabin outer shell/1 -> Integrator1/2
  Sum3/1 -> Product5/1
  area for heat transfer1/1 -> Product6/2
  heat transfer coefficient1/1 -> Product6/1
  Integrator1/1 -> Sum4/1, cabin outside shell temperature/1, Sum1/2, [tcabinshell]
  Sum4/1 -> Product6/3
  Product6/1 -> Sum/1, Mux/1, Sum3/2
  Sum5/1 -> Product2/1
  Product4/1 -> Sum5/2, Sum/3, Mux/3
  Lookup2/1 -> Mux1/2, Sum5/1
  Lookup1/1 -> Mux1/1, Sum3/3
  Mux1/1 -> solar heat flows/1
  Mux/1 -> cabin air heat transfer comps/1
  time1/1 -> Lookup2/1, Lookup1/1

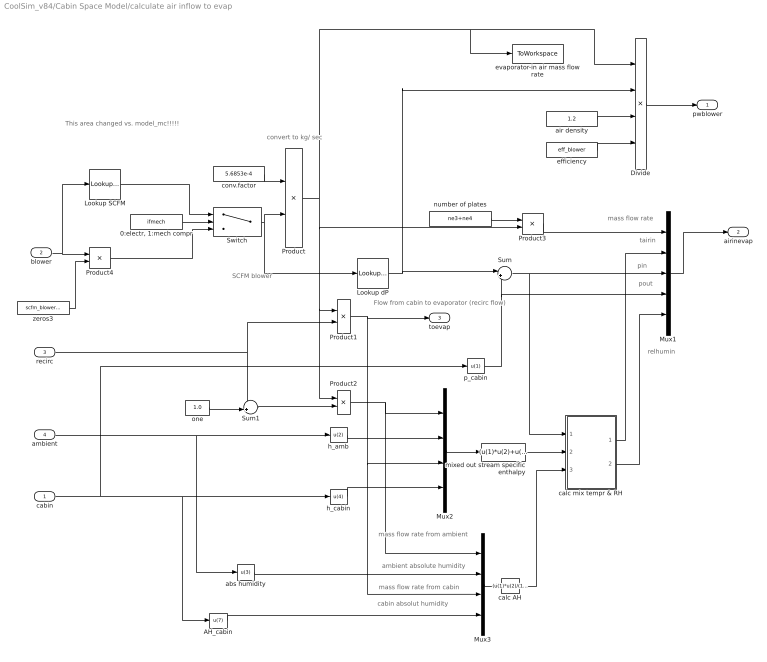
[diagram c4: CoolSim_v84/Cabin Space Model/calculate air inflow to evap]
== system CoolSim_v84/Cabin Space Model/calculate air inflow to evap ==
  note: mass flow rate
  note: tairin
  note: pin
  note: pout
  note: relhumin
  note: convert to kg/ sec
  note: Flow from cabin to evaporator (recirc flow)
  note: cabin absolut humidity
  note: ambient absolute humidity
  note: mass flow rate from ambient
  note: mass flow rate from cabin
  note: SCFM blower
  note: This area changed vs. model_mc!!!!!
  cabin : Inport
  blower : Inport  Port=2
  recirc : Inport  Port=3
  ambient : Inport  Port=4
  "0:electr, 1:mech compr" : Constant  Value=ifmech
  AH_cabin : Fcn  Expr=u(7)
  Divide : Product  Inputs=**//
  Lookup SCFM : Lookup_n-D  NumberOfTableDimensions=1  BreakpointsForDimension1=[0,1,2,3]  Table=scfm_blower  ExtrapMethod=Clip  RndMeth=Simplest
  Lookup dP : Lookup_n-D  NumberOfTableDimensions=1  BreakpointsForDimension1=scfm_blower  Table=dp_blower  ExtrapMethod=Clip  RndMeth=Simplest
  Mux1 : Mux  Inputs=5
  Mux2 : Mux
  Mux3 : Mux
  Product{,1..2,4} (4 alike) : Product
  Product3 : Product  Inputs=/*
  Sum : Sum  Inputs=|++
  Sum1 : Sum  Inputs=-+|
  Switch : Switch  Threshold=0.5
  abs humidity : Fcn  Expr=u(3)
  air density : Constant  Value=1.2
  calc AH : Fcn  Expr=(u(1)*u(2)/(1.+u(2))+u(3)*u(4)/(1.+u(4))) / (u(1)/(1.+u(2))+u(3)/(1.+u(4)))
  calc mix tempr & RH : Subsystem
  conv.factor : Constant  Value=5.6853e-4
  efficiency : Constant  Value=eff_blower
  evaporator-in air mass flow rate : ToWorkspace  VariableName=mdain_evap1  SampleTime=-1
  h_amb : Fcn  Expr=u(2)
  h_cabin : Fcn  Expr=u(4)
  mixed out stream specific enthalpy : Fcn  Expr=(u(1)*u(2)+u(3)*u(4))/(u(1)+u(3))
  number of plates : Constant  Value=ne3+ne4
  one : Constant  Value=1.0
  p_cabin : Fcn  Expr=u(1)
  zeros3 : Constant  Value=scfm_blower(4)
  pwblower : Outport
  airinevap : Outport  Port=2
  toevap : Outport  Port=3
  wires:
  cabin/1 -> h_cabin/1, AH_cabin/1, p_cabin/1
  recirc/1 -> Product1/2, Sum1/1
  ambient/1 -> abs humidity/1, h_amb/1
  mixed out stream specific enthalpy/1 -> calc mix tempr & RH/2(enth)
  Sum/1 -> Mux1/3, calc mix tempr & RH/1(press)
  Mux1/1 -> airinevap/1
  air density/1 -> Divide/3
  efficiency/1 -> Divide/4
  Divide/1 -> pwblower/1
  p_cabin/1 -> Mux1/4, Sum/2
  Lookup dP/1 -> Sum/1, Divide/2
  conv.factor/1 -> Product/1
  Product/1 -> evaporator-in air mass flow rate/1, Divide/1, Product1/1, Product2/1, Product3/2
  Product1/1 -> toevap/1, Mux3/3, Mux2/3
  one/1 -> Sum1/2
  h_cabin/1 -> Mux2/4
  Mux2/1 -> mixed out stream specific enthalpy/1
  Mux3/1 -> calc AH/1
  calc AH/1 -> calc mix tempr & RH/3(AH)
  calc mix tempr & RH/1(tempr) -> Mux1/2
  h_amb/1 -> Mux2/2
  calc mix tempr & RH/2(RH) -> Mux1/5
  AH_cabin/1 -> Mux3/4
  abs humidity/1 -> Mux3/2
  Sum1/1 -> Product2/2
  Product2/1 -> Mux2/1, Mux3/1
  Product3/1 -> Mux1/1
  number of plates/1 -> Product3/1
  zeros3/1 -> Product4/2
  blower/1 -> Product4/1, Lookup SCFM/1
  Switch/1 -> Product/2, Lookup dP/1
  "0:electr, 1:mech compr"/1 -> Switch/2
  Lookup SCFM/1 -> Switch/1
  Product4/1 -> Switch/3

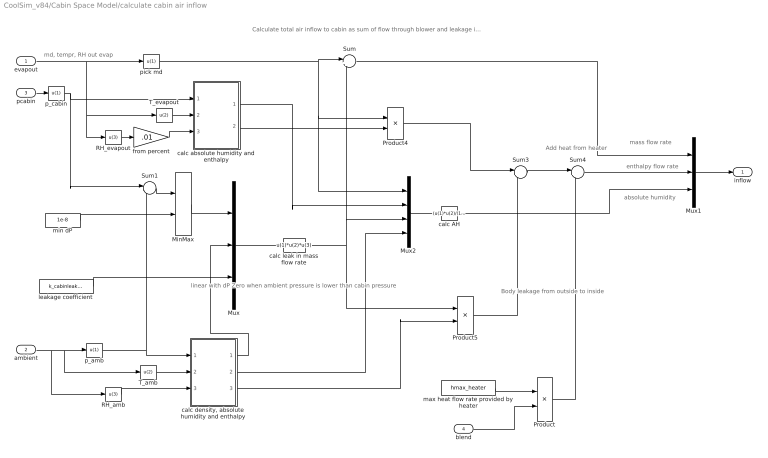
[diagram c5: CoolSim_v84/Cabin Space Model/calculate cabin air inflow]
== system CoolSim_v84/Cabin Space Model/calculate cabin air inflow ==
  note: Calculate total air inflow to cabin as sum of flow through blower and leakage into cabin from outside. Adjust enthalpy flow with heat added by heater
  note: md, tempr, RH out evap
  note: linear with dP Zero when ambient pressure is lower than cabin pressure
  note: absolute humidity
  note: mass flow rate
  note: enthalpy flow rate
  note: Add heat from heater
  note: Body leakage from outside to inside
  evapout : Inport
  ambient : Inport  Port=2
  pcabin : Inport  Port=3
  blend : Inport  Port=4
  MinMax : MinMax  Function=max  Inputs=2
  Mux : Mux  Inputs=3
  Mux1 : Mux  Inputs=3
  Mux2 : Mux
  Product : Product
  Product4 : Product
  Product5 : Product
  RH_amb : Fcn  Expr=u(3)
  RH_evapout : Fcn  Expr=u(3)
  Sum : Sum  Inputs=|++
  Sum1 : Sum  Inputs=|-+
  Sum3 : Sum  Inputs=|++
  Sum4 : Sum  Inputs=|++
  T_amb : Fcn  Expr=u(2)
  T_evapout : Fcn  Expr=u(2)
  calc AH : Fcn  Expr=(u(1)*u(2)/(1.+u(2))+u(3)*u(4)/(1.+u(4))) / (u(1)/(1.+u(2))+u(3)/(1.+u(4)))
  calc absolute humidity and enthalpy : Subsystem
  "calc density, absolute humidity and enthalpy" : Subsystem
  calc leak in mass flow rate : Fcn  Expr=u(1)*u(2)*u(3)
  from percent : Gain  Gain=.01
  leakage coefficient : Constant  Value=k_cabinleakin
  max heat flow rate provided by heater : Constant  Value=hmax_heater
  min dP : Constant  Value=1e-8
  p_amb : Fcn  Expr=u(1)
  p_cabin : Fcn  Expr=u(1)
  pick md : Fcn  Expr=u(1)
  inflow : Outport
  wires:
  evapout/1 -> T_evapout/1, RH_evapout/1, pick md/1
  blend/1 -> Product/2
  max heat flow rate provided by heater/1 -> Product/1
  pcabin/1 -> p_cabin/1
  T_evapout/1 -> calc absolute humidity and enthalpy/2(tempr)
  p_cabin/1 -> Sum1/1, calc absolute humidity and enthalpy/1(press)
  RH_evapout/1 -> from percent/1
  ambient/1 -> p_amb/1, T_amb/1, RH_amb/1
  p_amb/1 -> "calc density, absolute humidity and enthalpy"/1(press), Sum1/2
  T_amb/1 -> "calc density, absolute humidity and enthalpy"/2(tempr)
  RH_amb/1 -> "calc density, absolute humidity and enthalpy"/3(RH)
  calc leak in mass flow rate/1 -> Product5/1, Mux2/3, Sum/2
  Mux1/1 -> inflow/1
  Sum1/1 -> MinMax/1
  min dP/1 -> MinMax/2
  MinMax/1 -> Mux/1
  Mux/1 -> calc leak in mass flow rate/1
  Sum/1 -> Mux1/1
  calc absolute humidity and enthalpy/2(enth) -> Product4/2
  Product5/1 -> Sum3/2
  Product4/1 -> Sum3/1
  Sum4/1 -> Mux1/2
  Sum3/1 -> Sum4/1
  Product/1 -> Sum4/2
  "calc density, absolute humidity and enthalpy"/3(enth) -> Product5/2
  "calc density, absolute humidity and enthalpy"/1(dens) -> Mux/2
  calc absolute humidity and enthalpy/1(AH) -> Mux2/2
  "calc density, absolute humidity and enthalpy"/2(AH) -> Mux2/4
  Mux2/1 -> calc AH/1
  calc AH/1 -> Mux1/3
  leakage coefficient/1 -> Mux/3
  pick md/1 -> Sum/1, Product4/1, Mux2/1
  from percent/1 -> calc absolute humidity and enthalpy/3(RH)

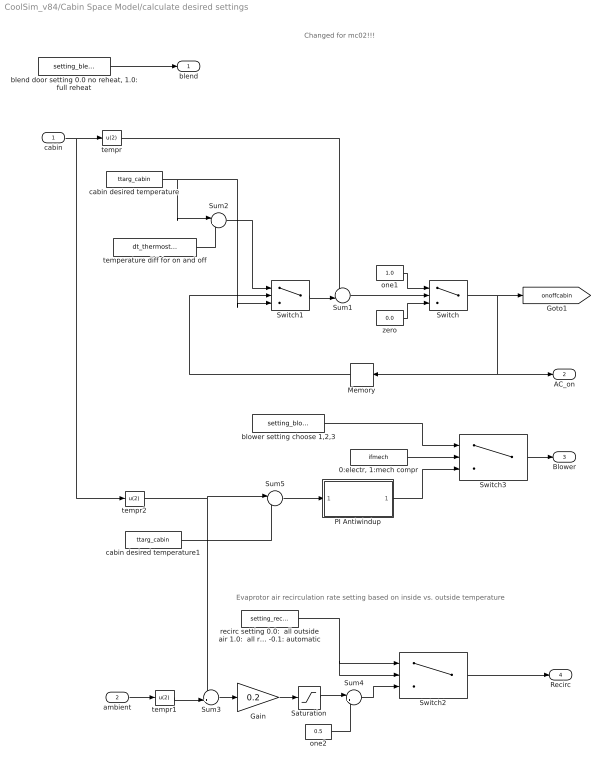
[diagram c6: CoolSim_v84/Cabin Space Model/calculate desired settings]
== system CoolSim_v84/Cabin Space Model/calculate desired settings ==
  note: Changed for mc02!!!
  note: Evaprotor air recirculation rate setting based on inside vs. outside temperature
  cabin : Inport
  ambient : Inport  Port=2
  "0:electr, 1:mech compr" : Constant  Value=ifmech
  Gain : Gain  Gain=0.2
  Memory : Memory  X0=onoffinit_cabin
  PI Antiwindup : Subsystem
  Saturation : Saturate  UpperLimit=0.45  LowerLimit=-0.45
  Sum1 : Sum  Inputs=+-|
  Sum2 : Sum  Inputs=|+-
  Sum3 : Sum  Inputs=-+|
  Sum4 : Sum  Inputs=|++
  Sum5 : Sum  Inputs=|-+
  Switch : Switch
  Switch1 : Switch  Threshold=0.5
  Switch2 : Switch  Threshold=-0.05
  Switch3 : Switch  Threshold=0.5
  "blend door setting 0.0 no reheat, 1.0: full reheat" : Constant  Value=setting_blend
  blower setting choose 1,2,3 : Constant  Value=setting_blower
  cabin desired temperature : Constant  Value=ttarg_cabin
  cabin desired temperature1 : Constant  Value=ttarg_cabin
  one1 : Constant  Value=1.0
  one2 : Constant  Value=0.5
  recirc setting 0.0:  all outside air 1.0:  all recirc air < -0.1: automatic : Constant  Value=setting_recirc
  temperature diff for on and off : Constant  Value=dt_thermostat
  tempr : Fcn  Expr=u(2)
  tempr1 : Fcn  Expr=u(2)
  tempr2 : Fcn  Expr=u(2)
  zero : Constant  Value=0.0
  blend : Outport
  AC_on : Outport  Port=2
  Blower : Outport  Port=3
  Recirc : Outport  Port=4
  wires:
  "0:electr, 1:mech compr"/1 -> Switch3/2
  cabin/1 -> tempr/1, tempr2/1
  "blend door setting 0.0 no reheat, 1.0: full reheat"/1 -> blend/1
  tempr/1 -> Sum1/1
  cabin desired temperature/1 -> Sum2/1, Switch1/3
  Sum2/1 -> Switch1/1
  Switch/1 -> Memory/1, AC_on/1, [onoffcabin]
  Sum1/1 -> Switch/2
  Switch1/1 -> Sum1/2
  Memory/1 -> Switch1/2
  one1/1 -> Switch/1
  zero/1 -> Switch/3
  temperature diff for on and off/1 -> Sum2/2
  Sum3/1 -> Gain/1
  recirc setting 0.0:  all outside air 1.0:  all recirc air < -0.1: automatic/1 -> Switch2/2, Switch2/1
  tempr1/1 -> Sum3/2
  ambient/1 -> tempr1/1
  Gain/1 -> Saturation/1
  Sum4/1 -> Switch2/3
  Saturation/1 -> Sum4/1
  one2/1 -> Sum4/2
  Switch2/1 -> Recirc/1
  tempr2/1 -> Sum5/1, Sum3/1
  cabin desired temperature1/1 -> Sum5/2
  Sum5/1 -> PI Antiwindup/1(err)
  blower setting choose 1,2,3/1 -> Switch3/1
  PI Antiwindup/1(cntrl) -> Switch3/3
  Switch3/1 -> Blower/1

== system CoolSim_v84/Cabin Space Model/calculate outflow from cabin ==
  note: Linear with dP Zero when ambient pressure is greater than cabin pressure
  note: md_out
  note: hd_out
  note: AH_out
  note: Calculate total air outflow from cabin, as the sum of recirc air outflow and leakage outflow
  cabin : Inport
  ambient : Inport  Port=2
  toevap : Inport  Port=3
  MinMax : MinMax  Function=max  Inputs=2
  Mux : Mux  Inputs=3
  Mux1 : Mux  Inputs=3
  Product1 : Product
  Sum : Sum  Inputs=|++
  Sum1 : Sum  Inputs=|+-
  calc leak out mass flow rate : Fcn  Expr=u(1)*u(2)*u(3)
  leakage effective flow area : Constant  Value=k_cabinleakout
  min dP : Constant  Value=1e-8
  pick AH : Fcn  Expr=u(7)
  pick density : Fcn  Expr=u(1)
  pick enthalpy : Fcn  Expr=u(4)
  pick press : Fcn  Expr=u(1)
  pick press1 : Fcn  Expr=u(1)
  outflow : Outport
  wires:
  cabin/1 -> pick enthalpy/1, pick AH/1, pick press/1
  ambient/1 -> pick press1/1
  calc leak out mass flow rate/1 -> Sum/2
  Sum/1 -> Product1/1, Mux1/1
  pick enthalpy/1 -> Product1/2
  Mux1/1 -> outflow/1
  Product1/1 -> Mux1/2
  pick AH/1 -> Mux1/3
  Sum1/1 -> MinMax/1
  min dP/1 -> MinMax/2
  MinMax/1 -> Mux/1
  Mux/1 -> calc leak out mass flow rate/1
  pick press/1 -> Sum1/1
  pick press1/1 -> Sum1/2
  toevap/1 -> Sum/1
  leakage effective flow area/1 -> Mux/3
  [ambextras] -> pick density/1
  pick density/1 -> Mux/2

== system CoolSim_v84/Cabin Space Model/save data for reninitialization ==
  onoff_cabin : Scope
  p_cabin : Scope
  picontr1 : Scope
  t_cabinint : Scope
  t_cabinshell : Scope
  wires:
  [pcabin] -> p_cabin/1
  [onoffcabin] -> onoff_cabin/1
  [tcabinint] -> t_cabinint/1
  [tcabinshell] -> t_cabinshell/1
  [picontr1] -> picontr1/1

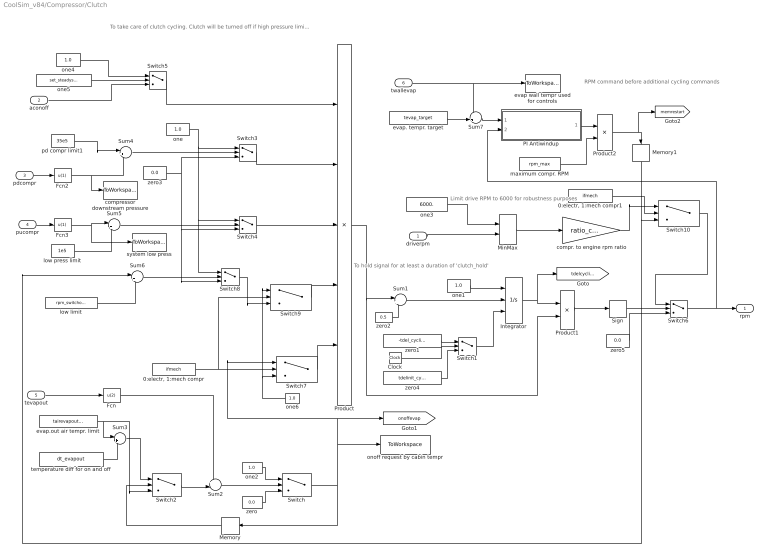
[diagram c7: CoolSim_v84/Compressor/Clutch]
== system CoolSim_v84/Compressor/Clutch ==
  note: To hold signal for at least a duration of 'clutch_hold'
  note: To take care of clutch cycling. Clutch will be turned off if high pressure limit, low pressure limit, or evaporator air temperature out low limit triggers it. It also turns off if temperature in the cabin drops below ttarg_cabin
  note: Limit drive RPM to 6000 for robustness purposes
  note: RPM command before additional cycling commands
  driverpm : Inport
  aconoff : Inport  Port=2
  pdcompr : Inport  Port=3
  pucompr : Inport  Port=4
  tevapout : Inport  Port=5
  twallevap : Inport  Port=6
  "0:electr, 1:mech compr" : Constant  Value=ifmech
  "0:electr, 1:mech compr1" : Constant  Value=ifmech
  Clock : Clock
  Fcn : Fcn  Expr=u(2)
  Fcn2 : Fcn  Expr=u(1)
  Fcn3 : Fcn  Expr=u(1)
  Integrator : Integrator  ExternalReset=falling  InitialConditionSource=external
  Memory : Memory  X0=onoffinit_evap
  Memory1 : Memory  X0=init_memrestart
  MinMax : MinMax  Inputs=2
  PI Antiwindup : Subsystem
  Product : Product  Inputs=5
  Product1 : Product
  Product2 : Product
  Sign : Signum
  Sum{1,3..6} (5 alike) : Sum  Inputs=|+-
  Sum2 : Sum  Inputs=+-|
  Sum7 : Sum  Inputs=-+|
  Switch : Switch
  Switch1 : Switch  Threshold=1e-8
  Switch{2,5..7,9..10} (6 alike) : Switch  Threshold=0.5
  Switch3 : Switch  Threshold=0.0
  Switch4 : Switch  Threshold=0.0
  Switch8 : Switch  Threshold=0.0
  compr. to engine rpm ratio : Gain  Gain=ratio_compr
  compressor downstream pressure : ToWorkspace  VariableName=pdcompr  SampleTime=-1
  evap wall tempr used for controls : ToWorkspace  VariableName=tevapwall  SampleTime=-1
  evap. tempr. target : Constant  Value=tevap_target
  evap.out air tempr. limit : Constant  Value=tairevapout_limit
  low limit : Constant  Value=rpm_switchoff
  low press limit : Constant  Value=1e5
  maximum compr. RPM : Constant  Value=rpm_max
  one{,1..2,4,6} (5 alike) : Constant  Value=1.0
  one3 : Constant  Value=6000.
  one5 : Constant  Value=set_steadystate
  onoff request by cabin tempr : ToWorkspace  VariableName=onoff_evap1  SampleTime=-1
  pd compr limit1 : Constant  Value=35e5
  system low press : ToWorkspace  VariableName=systplow  SampleTime=-1
  temperature diff for on and off : Constant  Value=dt_evapout
  zero : Constant  Value=0.0
  zero1 : Constant  Value=-tdel_cycling
  zero2 : Constant  Value=0.5
  zero3 : Constant  Value=0.0
  zero4 : Constant  Value=tdelinit_cycling
  zero5 : Constant  Value=0.0
  rpm : Outport
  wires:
  pd compr limit1/1 -> Sum4/1
  pdcompr/1 -> Fcn2/1
  Sum4/1 -> Switch3/2
  one/1 -> Switch3/1, Switch8/1, Switch4/1
  zero3/1 -> Switch3/3, Switch8/3, Switch4/3
  low press limit/1 -> Sum5/2
  pucompr/1 -> Fcn3/1
  Sum5/1 -> Switch4/2
  Switch3/1 -> Product/2
  Switch4/1 -> Product/3
  tevapout/1 -> Fcn/1
  Fcn/1 -> Sum2/1
  evap.out air tempr. limit/1 -> Sum3/1, Switch2/3
  Product/1 -> Sum1/1, Product1/2
  zero5/1 -> Switch6/3
  Switch6/1 -> rpm/1, PI Antiwindup/2(trig)
  one1/1 -> Integrator/1
  zero2/1 -> Sum1/2
  Sum1/1 -> Integrator/2
  Integrator/1 -> Product1/1, [tdelcycling]
  Product1/1 -> Sign/1
  Sign/1 -> Switch6/2
  zero1/1 -> Switch1/1
  Switch1/1 -> Integrator/3
  Clock/1 -> Switch1/2
  zero4/1 -> Switch1/3
  Sum3/1 -> Switch2/1
  Switch/1 -> Memory/1, [onoffevap], Switch7/1, onoff request by cabin tempr/1
  Sum2/1 -> Switch/2
  Switch2/1 -> Sum2/2
  Memory/1 -> Switch2/2
  one2/1 -> Switch/1
  zero/1 -> Switch/3
  temperature diff for on and off/1 -> Sum3/2
  driverpm/1 -> MinMax/2
  one3/1 -> MinMax/1
  one4/1 -> Switch5/1
  aconoff/1 -> Switch5/3
  one5/1 -> Switch5/2
  Switch5/1 -> Product/1
  MinMax/1 -> compr. to engine rpm ratio/1
  "0:electr, 1:mech compr"/1 -> Switch7/2, Switch9/2
  Switch7/1 -> Product/5
  one6/1 -> Switch7/3, Switch9/1
  low limit/1 -> Sum6/2
  Sum6/1 -> Switch8/2
  Switch9/1 -> Product/4
  Switch8/1 -> Switch9/3
  evap. tempr. target/1 -> Sum7/2
  PI Antiwindup/1(cntrl) -> Product2/1
  maximum compr. RPM/1 -> Product2/2
  twallevap/1 -> evap wall tempr used for controls/1, Sum7/1
  Sum7/1 -> PI Antiwindup/1(err)
  Product2/1 -> Memory1/1, [memrestart]
  Switch10/1 -> Switch6/1
  compr. to engine rpm ratio/1 -> Switch10/1
  Memory1/1 -> Switch10/3, Sum6/1
  "0:electr, 1:mech compr1"/1 -> Switch10/2
  Fcn2/1 -> Sum4/2, compressor downstream pressure/1
  Fcn3/1 -> Sum5/1, system low press/1

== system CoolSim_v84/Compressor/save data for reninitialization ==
  memrestart : Scope
  onoff_evap : Scope
  picontr2 : Scope
  tdel_cycling1 : Scope
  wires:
  [tdelcycling] -> tdel_cycling1/1
  [onoffevap] -> onoff_evap/1
  [picontr2] -> picontr2/1
  [memrestart] -> memrestart/1

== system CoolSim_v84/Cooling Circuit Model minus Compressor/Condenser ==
  ptrhu : Inport
  ptrhd : Inport  Port=2
  Gain : Gain  Gain=nc2
  Gain1 : Gain  Gain=nc1
  Gain2 : Gain  Gain=nc1
  Gain3 : Gain  Gain=nc1
  Gain4 : Gain  Gain=nc2
  Gain5 : Gain  Gain=nc2
  Integrator : Integrator
  R134a_line77_1 : Subsystem
  R134a_line77_2 : Subsystem
  R134a_volume11 condm1 : Subsystem
  Subtract : Sum
  condenser heat dumped to ambient : ToWorkspace  VariableName=qwr_cond  SampleTime=-1
  heat exchange : Constant  Value=0.0
  p_condm1 : Scope
  process incoming air conditions : Subsystem
  qwr_cond_scope : Scope
  volume2 : Constant  Value=[vol_condm1, 0]
  qmhu : Outport
  qmhd : Outport  Port=2
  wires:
  R134a_line77_1/2(qmhd) -> Gain3/1
  R134a_line77_1/1(qmhu) -> Gain1/1
  ptrhu/1 -> R134a_line77_1/1(pTrhu)
  heat exchange/1 -> R134a_volume11 condm1/3(Hout)
  volume2/1 -> R134a_volume11 condm1/2("V, dVdt")
  R134a_volume11 condm1/1(ptrh_mix) -> R134a_line77_2/1(pTrhu), p_condm1/1, [pcondm1], R134a_line77_1/2(pTrhd)
  R134a_line77_2/1(qmhu) -> Gain4/1
  R134a_line77_2/2(qmhd) -> Gain/1
  Gain/1 -> qmhd/1
  Gain1/1 -> qmhu/1
  [qwrcond1] -> Gain2/1
  [qwrcond2] -> Gain5/1
  Subtract/1 -> condenser heat dumped to ambient/1, Integrator/1
  ptrhd/1 -> R134a_line77_2/2(pTrhd)
  Gain3/1 -> R134a_volume11 condm1/1(qu)
  Gain4/1 -> R134a_volume11 condm1/4(qd)
  Gain2/1 -> Subtract/1
  Gain5/1 -> Subtract/2
  Integrator/1 -> qwr_cond_scope/1
